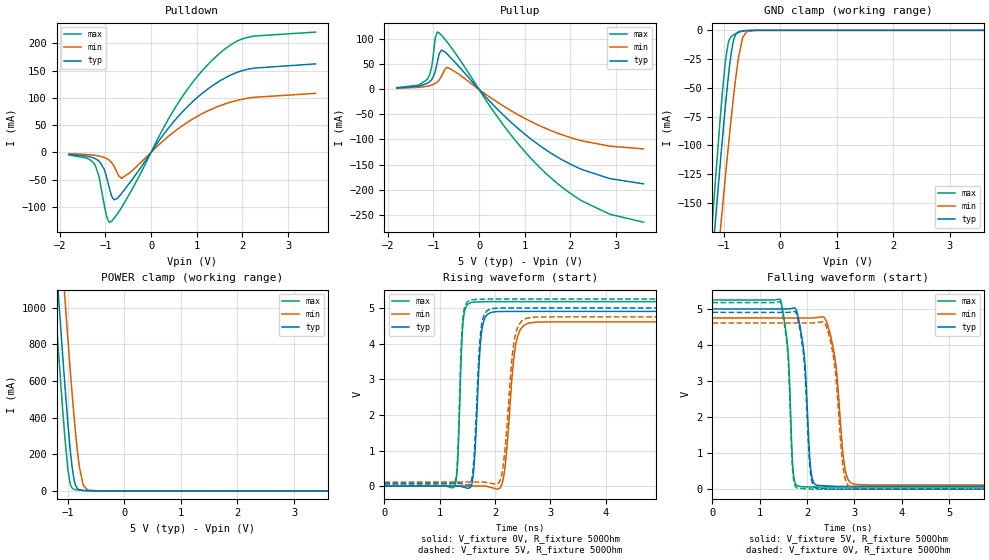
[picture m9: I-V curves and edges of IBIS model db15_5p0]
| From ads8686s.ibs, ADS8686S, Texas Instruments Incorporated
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|   db15_5p0 Model
[Model]   db15_5p0
Model_type   I/O
Polarity   Non-Inverting
Enable   Active-Low
Vinl = 1.5
Vinh = 3.5
Vmeas = 2.5
Vref = 2.5
Cref = 15pF
Rref = 50
|   typ   min   max
C_comp   1.49pF   1.49pF   1.52pF
[Voltage Range]   5   4.75   5.25
[Temperature Range]   27   125   -40
[Pullup Reference]   5   4.75   5.25
[Pulldown Reference]   0   0   0
[Power Clamp Reference]   5   4.75   5.25
[GND Clamp Reference]   0   0   0
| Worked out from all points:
|   slope of the pulldown table from 0 to 0.75 V, typ, clamps not added: 9.39 ohm
|   slope of the pullup table from 0 to 0.75 V, typ, clamps not added: 10.8 ohm
|   GND clamp passes 1 mA (typ) near -0.72 V on its own axis
|   POWER clamp passes 1 mA (typ) near -0.62 V on its own axis
|   falling waveform, V_fixture 5V, R_fixture 500Ohm: 20-80 % time 135ps typ, 190ps min, 111ps max; typ from 5 V to 0.078 V
|   rising waveform, V_fixture 0V, R_fixture 500Ohm: 20-80 % time 93.9ps typ, 142ps min, 68ps max; typ from 0 V to 4.9 V
|   rising waveform, V_fixture 5V, R_fixture 500Ohm: 20-80 % time 93.1ps typ, 143ps min, 66.5ps max; typ from 0.078 V to 5 V
|   falling waveform, V_fixture 0V, R_fixture 500Ohm: 20-80 % time 131ps typ, 180ps min, 109ps max; typ from 4.9 V to 0 V
[Pulldown]
|   Voltage   I(typ)   I(min)   I(max)
-1.8V     -3.825mA   -2.551mA   -4.908mA
-1.417V   -6.948mA   -4.028mA   -10.48mA
-1.233V   -11.26mA   -5.55mA    -22.46mA
-1.147V   -15.72mA   -6.73mA    -42.74mA
-979.2mV  -44mA      -11.19mA   -115.4mA
-876.6mV  -77.01mA   -17.72mA   -127.5mA
-806.4mV  -87.29mA   -26.35mA   -120.8mA
-649.8mV  -75.95mA   -47.84mA   -101.9mA
538.2mV   60.51mA    39.85mA    83.32mA
1.37V     123.9mA    80.83mA    171.8mA
2.126V    152.6mA    99.39mA    211.3mA
3.6V      162.3mA    108.2mA    220.8mA
[GND Clamp]
|   Voltage   I(typ)   I(min)   I(max)
-1.8V     -575.1mA   -590.1mA   -589.5mA
-1.211V   -205.2mA   -256.8mA   -174.1mA
-1.152V   -169.4mA   -224.2mA   -134.4mA
-1.066V   -118.7mA   -177.6mA   -79.19mA
-1.017V   -91.27mA   -151.8mA   -50.81mA
-963mV    -62.4mA    -123.9mA   -24.53mA
-903.6mV  -34.11mA   -94.13mA   -8.664mA
-822.6mV  -8.191mA   -56.42mA   -3.809mA
-736.2mV  -1.24mA    -23.24mA   -1.747mA
-666mV    -402uA     -6.834mA   -720.4uA
-595.8mV  -133uA     -1.235mA   -229.3uA
3.6V      0A         0A         0A
[Pullup]
|   Voltage   I(typ)   I(min)   I(max)
-1.8V     3.027mA    2.201mA    3.531mA
-1.136V   11.95mA    6.33mA     19.68mA
-1.044V   19mA       8.407mA    41.95mA
-957.6mV  36.26mA    11.91mA    102.1mA
-876.6mV  69.42mA    18.38mA    113.3mA
-822.6mV  78.66mA    26.06mA    108.3mA
-693mV    70.37mA    44.26mA    94.27mA
538.2mV   -51.62mA   -33.46mA   -71.85mA
1.445V    -119.6mA   -77.3mA    -166.1mA
2.261V    -160.3mA   -102.9mA   -223.1mA
2.887V    -178.5mA   -113.5mA   -249.9mA
3.6V      -188.6mA   -118.8mA   -265.2mA
[POWER Clamp]
|   Voltage   I(typ)   I(min)   I(max)
-1.8V     4.061A     4.54A      3.768A
-1.233V   1.367A     1.858A     1.061A
-1.179V   1.123A     1.613A     817.9mA
-1.049V   564.5mA    1.04A      280.1mA
-995.4mV  355.2mA    812.6mA    109.9mA
-963mV    243.1mA    681mA      46.78mA
-914.4mV  108.2mA    493.5mA    12.79mA
-865.8mV  32.73mA    323.4mA    7.075mA
-795.6mV  5.598mA    130.2mA    4.664mA
-730.8mV  2.41mA     35.35mA    3.08mA
-649.8mV  1.154mA    4.788mA    1.533mA
3.6V      0A         0A         0A
[Ramp]
R_load = 500
|   typ   min   max
dV/dt_r   2.94249/9.39205e-11   2.76609/1.42117e-10   3.10663/6.78166e-11
dV/dt_f   2.95306/1.35295e-10   2.78252/1.89222e-10   3.11407/1.10798e-10
[Falling Waveform]
V_fixture = 5V
V_fixture_min = 4.75V
V_fixture_max = 5.25V
R_fixture = 500Ohm
C_fixture = 0F
|   Time   V(typ)   V(min)   V(max)
0s        5V         4.75V      5.25V
1.437ns   4.999V     4.749V     5.258V
1.794ns   4.88V      4.749V     92.45mV
1.949ns   3.574V     4.749V     64.77mV
2.079ns   554.3mV    4.749V     61.01mV
2.198ns   112mV      4.761V     60.14mV
2.545ns   81.86mV    3.965V     60.13mV
2.773ns   78.52mV    813.3mV    60.12mV
2.946ns   78.51mV    160.2mV    60.12mV
10ns      78.24mV    112.5mV    59.88mV
[Rising Waveform]
V_fixture = 0V
V_fixture_min = 0V
V_fixture_max = 0V
R_fixture = 500Ohm
C_fixture = 0F
|   Time   V(typ)   V(min)   V(max)
0s        -62.79nV   -187.6nV   -117.4nV
1.265ns   3.703mV    2.97mV     -14.2mV
1.423ns   -25.08mV   3.341mV    4.629V
1.563ns   -11.9mV    3.669mV    5.155V
1.753ns   4.274V     4.115mV    5.172V
1.919ns   4.872V     -32.67mV   5.178V
2.139ns   4.901V     140mV      5.178V
2.369ns   4.904V     3.921V     5.178V
2.597ns   4.904V     4.569V     5.178V
10ns      4.904V     4.61V      5.178V
[Rising Waveform]
V_fixture = 5V
V_fixture_min = 4.75V
V_fixture_max = 5.25V
R_fixture = 500Ohm
C_fixture = 0F
|   Time   V(typ)   V(min)   V(max)
0s        78.24mV    112.5mV    59.88mV
1.265ns   81.84mV    115.3mV    54.39mV
1.417ns   58.53mV    115.6mV    4.677V
1.554ns   73.25mV    115.9mV    5.225V
1.745ns   4.393V     116.3mV    5.244V
1.912ns   4.969V     83.4mV     5.25V
2.118ns   4.997V     301.2mV    5.25V
2.343ns   5V         4.044V     5.25V
2.565ns   5V         4.708V     5.25V
10ns      5V         4.75V      5.25V
[Falling Waveform]
|Gnd
V_fixture = 0V
V_fixture_min = 0V
V_fixture_max = 0V
R_fixture = 500Ohm
C_fixture = 0F
|   Time   V(typ)   V(min)   V(max)
0s        4.904V     4.61V      5.178V
1.437ns   4.903V     4.609V     5.186V
1.594ns   4.903V     4.609V     3.732V
1.7ns     4.925V     4.609V     447.9mV
1.794ns   4.782V     4.609V     29.01mV
2.182ns   34.79mV    4.619V     241uV
2.502ns   2.785mV    4.055V     231.1uV
2.758ns   455.3uV    637.5mV    223.2uV
2.924ns   444.9uV    42.93mV    218.1uV
10ns      -14.41nV   8.141nV    -51.77nV
